(* Logix 5000 AddOnInstructionDefinition export EH_iTemp_TMT36_IOL; software revision 38.00 *)

TYPE EH_CommAOI_Data :
STRUCT
   Device_Comm_Error : BOOL;
   CommSuccess : BOOL;
   CommFailed : BOOL;
   CommTimeOut : BOOL;
   StateDone : BOOL;
   NewState : BOOL;
   OldState : SINT;
   PortSize : SINT;
   DevicePort : SINT;
   MaxState : SINT;
   State : SINT;
   VendorID : INT;
   DeviceID : DINT;
   CyclicData : INT[16];
   AcyclicData : DINT[8];
   ReplayIndex : INT;
   AOI_Diagnostic : DINT;
   ConnectionStatus : DINT;
   OutputData : INT[16];
END_STRUCT
END_TYPE

ADD_ON_INSTRUCTION EH_iTemp_TMT36_IOL   (* revision 1.1, vendor Endress+Hauser *)
// iTemp TMT36 Rev 1 IO-Link
// Revision note:
// 1.1 Changed the Datatype from Unsigned to Signed
// Add Disconnect check
VAR_IN_OUT
   DataToSend : INT[10]; {required}
   CommAOIBusy : DINT; {required}
   ActiveComPort : DINT; {required}
   DeviceAOISendRequest : DINT; {required}
   CommError : INT; {required}
   DeviceData : EH_CommAOI_Data; {required}
END_VAR
VAR_INPUT
   iSetSimulation : BOOL; {visible}
   iSimulationVariable : INT; {visible}
   iSimulationValue : REAL; {visible}
   iSetUnit : BOOL; {visible}
   iUnit : SINT; {visible}
   iParameterizeSetpoints : BOOL; {visible}
   iSSC1_SetPoint1 : REAL; {visible}
   iSSC1_SetPoint2 : REAL; {visible}
   iSSC1_Logic : SINT; {visible}
   iSSC1_Mode : SINT; {visible}
   iSSC1_Hysteresis : REAL; {visible}
   iSSC2_SetPoint1 : REAL; {visible}
   iSSC2_SetPoint2 : REAL; {visible}
   iSSC2_Logic : SINT; {visible}
   iSSC2_Mode : SINT; {visible}
   iSSC2_Hysteresis : REAL; {visible}
   iTeachSSC1 : BOOL; {visible}
   iSelectSP_SSC1 : SINT; {visible}
   iTeachSSC2 : BOOL; {visible}
   iSelectSP_SSC2 : SINT; {visible}
END_VAR
VAR_OUTPUT
   qVendor_ID : DINT; {access Read Only, visible}
   qDevice_ID : DINT; {access Read Only, visible}
   qTemperature : REAL; {visible}
   qExtendedDeviceStatus : INT; {access Read Only, visible}
   qSSC_1 : BOOL; {access Read Only, visible}
   qSSC1_SetPoint1 : REAL; {access Read Only, visible}
   qSSC1_SetPoint2 : REAL; {access Read Only, visible}
   qSSC_2 : BOOL; {access Read Only, visible}
   qSSC2_SetPoint1 : REAL; {access Read Only, visible}
   qSSC2_SetPoint2 : REAL; {access Read Only, visible}
   qUnit : DINT; {access Read Only, visible}
   qAOI_Diagnostic : DINT; {access Read Only, visible}
END_VAR
VAR_IN_OUT
   qAOI_Diagnostic_String : STRING; {required}
END_VAR
VAR_OUTPUT
   qActual_Diagnostics_Code : DINT; {access Read Only, visible}
END_VAR
VAR_IN_OUT
   qActual_Diagnostics_String : STRING; {required}
END_VAR
VAR_OUTPUT
   qLast_Diagnostics_Code : DINT; {visible}
END_VAR
VAR_IN_OUT
   qLast_Diagnostics_String : STRING; {required}
END_VAR
VAR_OUTPUT
   qCommError : DINT; {access None}
   qCommunicationBusy : DINT; {access Read Only, visible}
   qDeviceConnectionError : BOOL; {access Read Only, visible}
END_VAR
VAR
   Cond_DINT : DINT; {access None}
   Temp_DINT : DINT; {access None}
   Calc_Temperature : DINT; {access None}
   CMD_Index : INT; {access None}
   CMD_Subindex : INT; {access None}
   CMD_ByteLength : INT; {access None}
   oldCondStatus : INT; {access None}
   SetSimulation : SINT; {access None}
   SetTotalizer : SINT; {access None}
   oldSetSimulation : SINT; {access None}
   oldSetUnit : SINT; {access None}
   Trigger : BOOL; {access None}
   CMD_Rd : BOOL; {access None}
   CMD_Wr : BOOL; {access None}
   SimulationDINT : DINT; {access None}
   SimulationReal : DINT; {access None}
   Pressure_DINT : DINT; {access None}
   Level_DINT : DINT; {access None}
   InputByteLength : DINT; {access None}
   AOI_Prio : BOOL; {access None}
   ActiveAOI : BOOL; {access None}
   StateMin : DINT; {access None}
   firstTimeDone : BOOL; {access None}
   NextStep : BOOL; {access None}
   OldStatus : DINT; {access None}
   ChangedStatus : BOOL; {access None}
   CondStatusChanged : BOOL; {access None}
   Calc_ExtendedDeviceStatus : DINT; {access None}
   MassFlow_DINT : DINT; {access None}
   Density_DINT : DINT; {access None}
   oldParameterize : SINT; {access None}
   Parameterize : SINT; {access None}
   TeachSSC1Trigger : SINT; {access None}
   TeachSSC2Trigger : SINT; {access None}
   SimChanged : BOOL; {access None}
   Skip : BOOL; {access None}
   CondStatusActive : BOOL; {access None}
   SimActive : BOOL; {access None}
   DeviceID : DINT; {access None}
   FALSE : BOOL; {access None}
   TRUE : BOOL := 1; {access None}
   temp_string1 : STRING; {access None}
   temp_string2 : STRING; {access None}
   oldTeachSSC2Trigger : SINT; {access None}
   oldTeachSSC1Trigger : SINT; {access None}
   SetUnit : SINT; {access None}
   ParameterizeChanged : BOOL; {access None}
   ParameterizeActive : BOOL; {access None}
   TempAcyclic_DINT : DINT; {access None}
   TeachSSC2TriggerChanged : BOOL; {access None}
   TeachSSC1TriggerChanged : BOOL; {access None}
   TeachSSC1TriggerActive : BOOL; {access None}
   TeachSSC2TriggerActive : BOOL; {access None}
   StandardTimer : FBD_TIMER; {access None}
   qTemperatureTEMP : REAL; {access None}
   init : BOOL; {access None}
   UnitChanged : BOOL; {access None}
   UnitActive : BOOL; {access None}
END_VAR

ROUTINE Logic   (* structured text *)
// Picomag Communication via AL1323
   // =======================================================================
   // Endress+Hauser Digital Solutions
   // ©Copyright (2024) All Rights Reserved
   // =======================================================================
   // Name:                EH_iTemp_TMT36_IOL
   // Version:             1.1
   // Datum:               11.2025
   // Library:             01.01.00
   // Engineering:         Studio5000 V38.00.00
   // Author:              EH
   // =======================================================================
   
   qAOI_Diagnostic := DeviceData.AOI_Diagnostic;
   qCommunicationBusy := CommAOIBusy;
   DeviceID := 9698817;
   StateMin := 0;
   DeviceData.MaxState := 98;
   
   if DeviceData.DevicePort = 0 or DeviceData.DeviceID <> DeviceID or DeviceData.ConnectionStatus <> 1 then
   
   	qVendor_ID := DeviceData.VendorID;
   	qDevice_ID := DeviceData.DeviceID;
   	qTemperature	:= 0;
   	qExtendedDeviceStatus	:= 0;
   	qSSC_1	:= 0;
   	qSSC1_SetPoint1	:= 0;
   	qSSC1_SetPoint2	:= 0;
   	qSSC_2	:= 0;
   	qSSC2_SetPoint1	:= 0;
   	qSSC2_SetPoint2	:= 0;
   	qUnit := 0;
   	qActual_Diagnostics_Code	:= 0;
   	qLast_Diagnostics_Code	:= 0;
   	qLast_Diagnostics_String	:= '';
   	oldCondStatus := 0;
   	CondStatusChanged := FALSE;
   	init := FALSE;
   
   	if DeviceData.DevicePort = 0 then
   
   		qActual_Diagnostics_String	:= 'Device Port is Zero';
   		DeviceData.AOI_Diagnostic.1 := TRUE;
   
   	elsif DeviceData.ConnectionStatus <> 1 then
   
   		qActual_Diagnostics_String	:= 'No Device connected';
   		qDeviceConnectionError := TRUE;
   
   	elsif DeviceData.DeviceID <> DeviceID then
   
   		qActual_Diagnostics_String	:= 'Wrong DeviceID';
   		DeviceData.AOI_Diagnostic.2 := TRUE;
   	end_if;
   
   else
   
   	if qActual_Diagnostics_Code = 0  then
   
   		qActual_Diagnostics_String	:= '--------';
   
   	end_if;
   
   	if qLast_Diagnostics_Code = 0 then
   
   		qLast_Diagnostics_String	:= '--------';
   
   	end_if;
   
   	DeviceData.AOI_Diagnostic.1 := FALSE;
   	qDeviceConnectionError := FALSE;
   	DeviceData.AOI_Diagnostic.2  := FALSE;
   
   end_if;
   
   // Case device disconnected during communication to avoid blocking the communication
   if (DeviceData.AOI_Diagnostic.0 or qDeviceConnectionError or DeviceData.AOI_Diagnostic.2) and ActiveAOI and ActiveComPort = DeviceData.DevicePort and CommAOIBusy = 1 then
   
   	DeviceData.State := 0;
   	CommAOIBusy := 0;
   	DeviceAOISendRequest.[DeviceData.DevicePort] := 0;
   	ActiveComPort := 0;
   	ActiveAOI := 0;
   	DataToSend[0] := 0;
   	DataToSend[1] := 0;
   	DataToSend[2] := 0;
   	DataToSend[3] := 0;
   	DataToSend[4] := 0;
   	DataToSend[5] := 0;
   	DataToSend[6] := 0;
   	DataToSend[7] := 0;
   	DataToSend[8] := 0;
   	DataToSend[9] := 0;
   	DeviceData.StateDone := FALSE;
   	DeviceData.NewState := FALSE;
   	DeviceData.OldState := 0;
   	ActiveAOI := FALSE;
   
   end_if;
   
   if not DeviceData.AOI_Diagnostic.0
   	and not qDeviceConnectionError
   	and not DeviceData.AOI_Diagnostic.2
   	and DeviceData.DevicePort > 0 then
   
   	//*********************************
   	//Vendor ID
   	//*********************************
   
   		qVendor_ID := DeviceData.VendorID;
   
   	//*********************************
   	//Device ID
   	//*********************************
   
   		qDevice_ID := DeviceData.DeviceID;
   
   	//*********************************
   	// TMT36 Cyclic Input
   	//*********************************
   
   		Calc_Temperature			:= 0;
   		Calc_ExtendedDeviceStatus	:= 2;
   
   	//*********************************
   	//Process Data Temperature
   	//*********************************
   
   		Temp_DINT	 := DeviceData.CyclicData[Calc_Temperature+1];
   		Temp_DINT.8	 := DeviceData.CyclicData[Calc_Temperature+1].8;
   		Temp_DINT.9  := DeviceData.CyclicData[Calc_Temperature+1].9;
   		Temp_DINT.10 := DeviceData.CyclicData[Calc_Temperature+1].10;
   		Temp_DINT.11 := DeviceData.CyclicData[Calc_Temperature+1].11;
   		Temp_DINT.12 := DeviceData.CyclicData[Calc_Temperature+1].12;
   		Temp_DINT.13 := DeviceData.CyclicData[Calc_Temperature+1].13;
   		Temp_DINT.14 := DeviceData.CyclicData[Calc_Temperature+1].14;
   		Temp_DINT.15 := DeviceData.CyclicData[Calc_Temperature+1].15;
   		Temp_DINT.16 := DeviceData.CyclicData[Calc_Temperature].0;
   		Temp_DINT.17 := DeviceData.CyclicData[Calc_Temperature].1;
   		Temp_DINT.18 := DeviceData.CyclicData[Calc_Temperature].2;
   		Temp_DINT.19 := DeviceData.CyclicData[Calc_Temperature].3;
   		Temp_DINT.20 := DeviceData.CyclicData[Calc_Temperature].4;
   		Temp_DINT.21 := DeviceData.CyclicData[Calc_Temperature].5;
   		Temp_DINT.22 := DeviceData.CyclicData[Calc_Temperature].6;
   		Temp_DINT.23 := DeviceData.CyclicData[Calc_Temperature].7;
   		Temp_DINT.24 := DeviceData.CyclicData[Calc_Temperature].8;
   		Temp_DINT.25 := DeviceData.CyclicData[Calc_Temperature].9;
   		Temp_DINT.26 := DeviceData.CyclicData[Calc_Temperature].10;
   		Temp_DINT.27 := DeviceData.CyclicData[Calc_Temperature].11;
   		Temp_DINT.28 := DeviceData.CyclicData[Calc_Temperature].12;
   		Temp_DINT.29 := DeviceData.CyclicData[Calc_Temperature].13;
   		Temp_DINT.30 := DeviceData.CyclicData[Calc_Temperature].14;
   		Temp_DINT.31 := DeviceData.CyclicData[Calc_Temperature].15;
   
   		COP(Temp_DINT,qTemperatureTEMP,1);
   
   		// Unit of the process value, 32 = °C, 33 = °F
   		if qUnit = 33 then
   
   			qTemperature := (qTemperatureTEMP * 1.8) +32;
   
   		else
   
   			qTemperature := qTemperatureTEMP;
   
   		end_if;
   
   
   	//*********************************
   	// Extended device Status
   	//*********************************
   
   		qExtendedDeviceStatus.0 := DeviceData.CyclicData[Calc_ExtendedDeviceStatus].8;
   		qExtendedDeviceStatus.1 := DeviceData.CyclicData[Calc_ExtendedDeviceStatus].9;
   		qExtendedDeviceStatus.2 := DeviceData.CyclicData[Calc_ExtendedDeviceStatus].10;
   		qExtendedDeviceStatus.3 := DeviceData.CyclicData[Calc_ExtendedDeviceStatus].11;
   		qExtendedDeviceStatus.4 := DeviceData.CyclicData[Calc_ExtendedDeviceStatus].12;
   		qExtendedDeviceStatus.5 := DeviceData.CyclicData[Calc_ExtendedDeviceStatus].13;
   		qExtendedDeviceStatus.6 := DeviceData.CyclicData[Calc_ExtendedDeviceStatus].14;
   		qExtendedDeviceStatus.7 := DeviceData.CyclicData[Calc_ExtendedDeviceStatus].15;
   
   	//*********************************
   	// Process Parameter SSC
   	//*********************************
   
   		qSSC_1 := DeviceData.CyclicData[Calc_ExtendedDeviceStatus].0;
   		qSSC_2 := DeviceData.CyclicData[Calc_ExtendedDeviceStatus].1;
   
   	//*********************************
   	// Checking for Changed Status @ Input or Condenced Status
   	//*********************************
   
   	SetSimulation.0 := iSetSimulation;
   	Parameterize.0 := iParameterizeSetpoints;
   	TeachSSC1Trigger.0 := iTeachSSC1;
   	TeachSSC2Trigger.0 := iTeachSSC2;
   	SetUnit.0 := iSetUnit;
   
   	if oldCondStatus <> qExtendedDeviceStatus and not CondStatusChanged then
   
   		CondStatusChanged := TRUE;
   		oldCondStatus := qExtendedDeviceStatus;
   
   	end_if;
   
   	if oldSetSimulation <> SetSimulation and not SimChanged then
   
   		if oldSetSimulation < SetSimulation then
   
   			SimChanged := TRUE;
   
   		end_if;
   
   		oldSetSimulation := SetSimulation;
   
   	end_if;
   
   	if oldSetUnit <> SetUnit and not UnitChanged then
   
   		if oldSetUnit < SetUnit then
   
   			UnitChanged := TRUE;
   
   		end_if;
   
   		oldSetUnit := SetUnit;
   
   	end_if;
   
   	if oldParameterize <> Parameterize and not ParameterizeChanged then
   
   		if oldParameterize < Parameterize then
   
   			ParameterizeChanged := TRUE;
   
   		end_if;
   
   		oldParameterize := Parameterize;
   
   	end_if;
   
   	if oldTeachSSC1Trigger <> TeachSSC1Trigger and not TeachSSC1TriggerChanged then
   
   		if oldTeachSSC1Trigger < TeachSSC1Trigger then
   
   			TeachSSC1TriggerChanged := TRUE;
   
   		end_if;
   
   		oldTeachSSC1Trigger := TeachSSC1Trigger;
   
   	end_if;
   
   	if oldTeachSSC2Trigger <> TeachSSC2Trigger and not TeachSSC2TriggerChanged then
   
   		if oldTeachSSC2Trigger < TeachSSC2Trigger then
   
   			TeachSSC2TriggerChanged := TRUE;
   
   		end_if;
   
   		oldTeachSSC2Trigger := TeachSSC2Trigger;
   
   	end_if;
   
   	if CondStatusChanged
   	and not ActiveAOI
   	and not CondStatusActive
   	and not Skip then
   
   		DeviceAOISendRequest.[DeviceData.DevicePort] := TRUE;
   		CondStatusActive := TRUE;
   		Skip := TRUE;
   
   	elsif SimChanged
   		and not ActiveAOI
   		and not SimActive
   		and not Skip then
   
   		DeviceAOISendRequest.[DeviceData.DevicePort] := TRUE;
   		SimActive := TRUE;
   		Skip := TRUE;
   
   	elsif UnitChanged
   		and not ActiveAOI
   		and not UnitActive
   		and not Skip then
   
   		DeviceAOISendRequest.[DeviceData.DevicePort] := TRUE;
   		UnitActive := TRUE;
   		Skip := TRUE;
   
   	elsif TeachSSC1TriggerChanged
   		and not ActiveAOI
   		and not TeachSSC1TriggerActive
   		and not Skip then
   
   		DeviceAOISendRequest.[DeviceData.DevicePort] := TRUE;
   		TeachSSC1TriggerActive := TRUE;
   		Skip := TRUE;
   
   	elsif TeachSSC2TriggerChanged
   		and not ActiveAOI
   		and not TeachSSC2TriggerActive
   		and not Skip then
   
   		DeviceAOISendRequest.[DeviceData.DevicePort] := TRUE;
   		TeachSSC2TriggerActive := TRUE;
   		Skip := TRUE;
   
   	elsif ParameterizeChanged
   		and not ActiveAOI
   		and not ParameterizeActive
   		and not Skip then
   
   		DeviceAOISendRequest.[DeviceData.DevicePort] := TRUE;
   		ParameterizeActive := TRUE;
   		Skip := TRUE;
   
   	end_if;
   
   	if ActiveComPort = DeviceData.DevicePort then
   
   		AOI_Prio := TRUE;
   
   	else
   
   		AOI_Prio := FALSE;
   
   	end_if;
   
   	if (SimActive or UnitActive or TeachSSC1TriggerActive or TeachSSC2TriggerActive or ParameterizeActive or CondStatusActive) and CommAOIBusy = 1  and DeviceData.State = 0 and AOI_Prio and not ActiveAOI then
   
   		ActiveAOI := TRUE;
   		Skip := FALSE;
   
   	end_if;
   
   	qCommunicationBusy := CommAOIBusy;
   	qAOI_Diagnostic :=DeviceData.AOI_Diagnostic;
   
   	//*********************************
   	// States for Execution
   	//*********************************
   
   	if ActiveAOI or DeviceData.State = DeviceData.MaxState then
   
   	case DeviceData.State of
   
   		//*********************************
   		0: // Start
   		//*********************************
   
   			Trigger := FALSE;
   			CMD_Index := 0;
   			CMD_Subindex := 0;
   			CMD_Wr := FALSE;
   			CMD_Rd := FALSE;
   			CMD_ByteLength := 0;
   
   			if DeviceData.DevicePort = ActiveComPort then
   
   				DeviceData.CommSuccess := FALSE;
   				DeviceData.CommTimeOut := FALSE;
   				DeviceData.NewState := TRUE;
   				DeviceData.StateDone := FALSE;
   
   			end_if;
   
   			if SimActive then
   
   				DeviceData.AOI_Diagnostic := 0;
   				DeviceData.State := 1;
   
   			elsif UnitActive then
   
   				DeviceData.AOI_Diagnostic := 0;
   				DeviceData.State := 4;
   
   			elsif ParameterizeActive then
   
   				DeviceData.AOI_Diagnostic := 0;
   				DeviceData.State := 43;
   
   			elsif TeachSSC1TriggerActive then
   
   				DeviceData.AOI_Diagnostic := 0;
   				DeviceData.State := 50;
   
   			elsif TeachSSC2TriggerActive then
   
   				DeviceData.AOI_Diagnostic := 0;
   				DeviceData.State := 60;
   
   			elsif CondStatusChanged then
   
   				if not init then
   
   					DeviceData.State := 5;
   
   				else
   
   					DeviceData.State := 90;
   
   				end_if;
   
   			end_if;
   
   		//*********************************
   		1: // Set Simulation
   		//*********************************
   
   			CMD_Index := 8259;
   			CMD_Subindex := 0;
   			CMD_Wr := TRUE;	// Only Read or Write can be active
   			CMD_Rd := FALSE;
   			CMD_ByteLength := 1;	//Check Length
   			DataToSend[6]:= 0;
   			DataToSend[7]:= 0;
   
   			// 0 = Off, 1 = Temperature
   			DataToSend[6].0 := iSimulationVariable.0;
   			DataToSend[6].1 := iSimulationVariable.1;
   			DataToSend[6].2 := iSimulationVariable.2;
   			DataToSend[6].3 := iSimulationVariable.3;
   			DataToSend[6].4 := iSimulationVariable.4;
   			DataToSend[6].5 := iSimulationVariable.5;
   			DataToSend[6].6 := iSimulationVariable.6;
   			DataToSend[6].7 := iSimulationVariable.7;
   
   			Trigger := TRUE;
   
   			if DeviceData.NewState then
   
   				DeviceData.StateDone := TRUE;
   
   			end_if;
   
   			if  DeviceData.CommSuccess and DeviceData.ReplayIndex = CMD_Index then
   
   				Trigger := FALSE;
   				DeviceData.OldState := DeviceData.State;
   				DeviceData.State := DeviceData.State + 1;
   				DeviceData.CommSuccess := FALSE;
   				DeviceData.AcyclicData[0] := 0;
   				DeviceData.NewState := TRUE;
   
   			elsif DeviceData.CommTimeOut then
   
   				temp_string1 := 'Error in step ';
   				Temp_DINT := DeviceData.State;
   				DTOS(Temp_DINT, temp_string2);
   				CONCAT(temp_string1, temp_string2, qAOI_Diagnostic_String);
   
   				DeviceData.OldState := DeviceData.State;
   				DeviceData.State := DeviceData.MaxState;
   				DeviceData.CommTimeOut := FALSE;
   				DeviceData.AcyclicData[0] := 0;
   				DeviceData.NewState := TRUE;
   
   			end_if;
   
   
   		//*********************************
   		2: // Set Simulation Value
   		//*********************************
   
   			CMD_Index := 8254;
   			CMD_Subindex := 0;
   			CMD_Wr := TRUE;
   			CMD_Rd := FALSE;
   			CMD_ByteLength := 4;
   			DataToSend[6]:= 0;
   			DataToSend[7]:= 0;
   
   		 	COP(iSimulationValue,SimulationDINT,1);		// Copy the Bits from the Real in a DINT
   
   			DataToSend[6].0 :=  SimulationDINT.24;
   			DataToSend[6].1 :=  SimulationDINT.25;
   			DataToSend[6].2 :=  SimulationDINT.26;
   			DataToSend[6].3 :=  SimulationDINT.27;
   			DataToSend[6].4 :=  SimulationDINT.28;
   			DataToSend[6].5 :=  SimulationDINT.29;
   			DataToSend[6].6 :=  SimulationDINT.30;
   			DataToSend[6].7 :=  SimulationDINT.31;
   			DataToSend[6].8 :=  SimulationDINT.16;
   			DataToSend[6].9 :=  SimulationDINT.17;
   			DataToSend[6].10 := SimulationDINT.18;
   			DataToSend[6].11 := SimulationDINT.19;
   			DataToSend[6].12 := SimulationDINT.20;
   			DataToSend[6].13 := SimulationDINT.21;
   			DataToSend[6].14 := SimulationDINT.22;
   			DataToSend[6].15 := SimulationDINT.23;
   			DataToSend[7].0  := SimulationDINT.8;
   			DataToSend[7].1  := SimulationDINT.9;
   			DataToSend[7].2  := SimulationDINT.10;
   			DataToSend[7].3  := SimulationDINT.11;
   			DataToSend[7].4  := SimulationDINT.12;
   			DataToSend[7].5  := SimulationDINT.13;
   			DataToSend[7].6  := SimulationDINT.14;
   			DataToSend[7].7  := SimulationDINT.15;
   			DataToSend[7].8  := SimulationDINT.0;
   			DataToSend[7].9  := SimulationDINT.1;
   			DataToSend[7].10 := SimulationDINT.2;
   			DataToSend[7].11 := SimulationDINT.3;
   			DataToSend[7].12 := SimulationDINT.4;
   			DataToSend[7].13 := SimulationDINT.5;
   			DataToSend[7].14 := SimulationDINT.6;
   			DataToSend[7].15 := SimulationDINT.7;
   
   			Trigger := TRUE;
   
   			if DeviceData.NewState then
   
   				DeviceData.StateDone := TRUE;
   
   			end_if;
   
   			if DeviceData.CommSuccess and DeviceData.ReplayIndex = CMD_Index then
   
   				Trigger := FALSE;
   				DeviceData.OldState := DeviceData.State;
   				DeviceData.State := DeviceData.MaxState;
   				DeviceData.CommSuccess := FALSE;
   				DeviceData.AcyclicData[0] := 0;
   				DeviceData.NewState := TRUE;
   
   			elsif DeviceData.CommTimeOut then
   
   				temp_string1 := 'Error in step ';
   				Temp_DINT := DeviceData.State;
   				DTOS(Temp_DINT, temp_string2);
   				CONCAT(temp_string1, temp_string2, qAOI_Diagnostic_String);
   
   				DeviceData.OldState := DeviceData.State;
   				DeviceData.State := DeviceData.MaxState;	//Check State
   				DeviceData.CommTimeOut := FALSE;
   				DeviceData.AcyclicData[0] := 0;
   				DeviceData.NewState := TRUE;
   
   			end_if;
   
   		//*********************************
   		4: // Set Unit
   		//*********************************
   
   			CMD_Index := 8274;
   			CMD_Subindex := 0;
   			CMD_Wr := TRUE;								// Only Read or Write can be active = 1
   			CMD_Rd := FALSE;
   			CMD_ByteLength := 1;
   			DataToSend[6] := 0;
   			DataToSend[7] := 0;
   
   			if iUnit = 32 OR iUnit = 33 then
   
   				DataToSend[6].0 := iUnit.0;
   				DataToSend[6].1 := iUnit.1;
   				DataToSend[6].2 := iUnit.2;
   				DataToSend[6].3 := iUnit.3;
   				DataToSend[6].4 := iUnit.4;
   				DataToSend[6].5 := iUnit.5;
   				DataToSend[6].6 := iUnit.6;
   				DataToSend[6].7 := iUnit.7;
   				Trigger := TRUE;
   
   				if DeviceData.NewState then
   					DeviceData.StateDone := TRUE;
   				end_if;
   
   				if  DeviceData.CommSuccess and DeviceData.ReplayIndex = CMD_Index then
   
   					Trigger := FALSE;
   					DeviceData.OldState := DeviceData.State;
   					DeviceData.State := DeviceData.State + 1;
   					DeviceData.CommSuccess := FALSE;
   					DeviceData.AcyclicData[0] := 0;
   					DeviceData.NewState := TRUE;
   
   			 	elsif DeviceData.CommTimeOut then
   
   					temp_string1 := 'Error in step ';
   					Temp_DINT := DeviceData.State;
   					DTOS(Temp_DINT, temp_string2);
   					CONCAT(temp_string1, temp_string2, qAOI_Diagnostic_String);
   
   					DeviceData.OldState := DeviceData.State;
   					DeviceData.State := DeviceData.MaxState;	//Check State
   					DeviceData.CommTimeOut := FALSE;
   					DeviceData.AcyclicData[0] := 0;
   					DeviceData.NewState := TRUE;
   
   				end_if;
   
   			else
   
   					temp_string1 := 'Error in step ';
   					Temp_DINT := DeviceData.State;
   					DTOS(Temp_DINT, temp_string2);
   					CONCAT(temp_string1, temp_string2, qAOI_Diagnostic_String);
   
   					DeviceData.OldState := DeviceData.State;
   					DeviceData.State := DeviceData.MaxState;
   					DeviceData.CommTimeOut := FALSE;
   					DeviceData.AcyclicData[0] := 0;
   					DeviceData.NewState := TRUE;
   
   	        end_if;
   
   
   		//*********************************
   		5: // Read Unit
   		//*********************************
   
   				CMD_Index := 8274;
   				CMD_Subindex := 0;
   				CMD_Wr := FALSE;
   				CMD_Rd := TRUE;
   				CMD_ByteLength := 1;
   				Trigger := TRUE;
   
   				if DeviceData.NewState then
   					DeviceData.StateDone := TRUE;
   				end_if;
   
   				if  DeviceData.CommSuccess and DeviceData.ReplayIndex = CMD_Index then
   
   					qUnit.0	:= DeviceData.AcyclicData[0].0;
   					qUnit.1	:= DeviceData.AcyclicData[0].1;
   					qUnit.2	:= DeviceData.AcyclicData[0].2;
   					qUnit.3	:= DeviceData.AcyclicData[0].3;
   					qUnit.4	:= DeviceData.AcyclicData[0].4;
   					qUnit.5	:= DeviceData.AcyclicData[0].5;
   					qUnit.6	:= DeviceData.AcyclicData[0].6;
   					qUnit.7	:= DeviceData.AcyclicData[0].7;
   
   					Trigger := FALSE;
   					DeviceData.OldState := DeviceData.State;
   					DeviceData.State := DeviceData.MaxState;
   					DeviceData.CommSuccess := FALSE;
   					DeviceData.AcyclicData[0] := 0;
   					DeviceData.NewState := TRUE;
   
   					if not init then
   
   						init := TRUE;
   						DeviceData.State := 90;
   
   					end_if;
   
   				 elsif DeviceData.CommTimeOut then
   
   					temp_string1 := 'Error in step ';
   					Temp_DINT := DeviceData.State;
   					DTOS(Temp_DINT, temp_string2);
   					CONCAT(temp_string1, temp_string2, qAOI_Diagnostic_String);
   
   					DeviceData.OldState := DeviceData.State;
   					DeviceData.State := DeviceData.MaxState;
   					DeviceData.CommTimeOut := FALSE;
   					DeviceData.AcyclicData[0] := 0;
   					DeviceData.NewState := TRUE;
   
   				end_if;
   
   
   		//************************************
   		43: // SSC1 Setpoint - SSC1 param
   		//************************************
   
   			CMD_Index := 60;
   			CMD_Subindex := 0;
   			CMD_Wr := TRUE;
   			CMD_Rd := FALSE;
   			CMD_ByteLength := 8;
   			DataToSend[6]:= 0;
   			DataToSend[7]:= 0;
   			DataToSend[8]:= 0;
   			DataToSend[9]:= 0;
   
   		 	COP(iSSC1_SetPoint1,SimulationDINT,1);		// Copy the Bits from the Real in a DINT
   
   			DataToSend[6].0 :=  SimulationDINT.24;
   			DataToSend[6].1 :=  SimulationDINT.25;
   			DataToSend[6].2 :=  SimulationDINT.26;
   			DataToSend[6].3 :=  SimulationDINT.27;
   			DataToSend[6].4 :=  SimulationDINT.28;
   			DataToSend[6].5 :=  SimulationDINT.29;
   			DataToSend[6].6 :=  SimulationDINT.30;
   			DataToSend[6].7 :=  SimulationDINT.31;
   			DataToSend[6].8 :=  SimulationDINT.16;
   			DataToSend[6].9 :=  SimulationDINT.17;
   			DataToSend[6].10 := SimulationDINT.18;
   			DataToSend[6].11 := SimulationDINT.19;
   			DataToSend[6].12 := SimulationDINT.20;
   			DataToSend[6].13 := SimulationDINT.21;
   			DataToSend[6].14 := SimulationDINT.22;
   			DataToSend[6].15 := SimulationDINT.23;
   			DataToSend[7].0  := SimulationDINT.8;
   			DataToSend[7].1  := SimulationDINT.9;
   			DataToSend[7].2  := SimulationDINT.10;
   			DataToSend[7].3  := SimulationDINT.11;
   			DataToSend[7].4  := SimulationDINT.12;
   			DataToSend[7].5  := SimulationDINT.13;
   			DataToSend[7].6  := SimulationDINT.14;
   			DataToSend[7].7  := SimulationDINT.15;
   			DataToSend[7].8  := SimulationDINT.0;
   			DataToSend[7].9  := SimulationDINT.1;
   			DataToSend[7].10 := SimulationDINT.2;
   			DataToSend[7].11 := SimulationDINT.3;
   			DataToSend[7].12 := SimulationDINT.4;
   			DataToSend[7].13 := SimulationDINT.5;
   			DataToSend[7].14 := SimulationDINT.6;
   			DataToSend[7].15 := SimulationDINT.7;
   
   			COP(iSSC1_SetPoint2,SimulationDINT,1);		// Copy the Bits from the Real in a DINT
   
   			DataToSend[8].0 :=  SimulationDINT.24;
   			DataToSend[8].1 :=  SimulationDINT.25;
   			DataToSend[8].2 :=  SimulationDINT.26;
   			DataToSend[8].3 :=  SimulationDINT.27;
   			DataToSend[8].4 :=  SimulationDINT.28;
   			DataToSend[8].5 :=  SimulationDINT.29;
   			DataToSend[8].6 :=  SimulationDINT.30;
   			DataToSend[8].7 :=  SimulationDINT.31;
   			DataToSend[8].8 :=  SimulationDINT.16;
   			DataToSend[8].9 :=  SimulationDINT.17;
   			DataToSend[8].10 := SimulationDINT.18;
   			DataToSend[8].11 := SimulationDINT.19;
   			DataToSend[8].12 := SimulationDINT.20;
   			DataToSend[8].13 := SimulationDINT.21;
   			DataToSend[8].14 := SimulationDINT.22;
   			DataToSend[8].15 := SimulationDINT.23;
   			DataToSend[9].0  := SimulationDINT.8;
   			DataToSend[9].1  := SimulationDINT.9;
   			DataToSend[9].2  := SimulationDINT.10;
   			DataToSend[9].3  := SimulationDINT.11;
   			DataToSend[9].4  := SimulationDINT.12;
   			DataToSend[9].5  := SimulationDINT.13;
   			DataToSend[9].6  := SimulationDINT.14;
   			DataToSend[9].7  := SimulationDINT.15;
   			DataToSend[9].8  := SimulationDINT.0;
   			DataToSend[9].9  := SimulationDINT.1;
   			DataToSend[9].10 := SimulationDINT.2;
   			DataToSend[9].11 := SimulationDINT.3;
   			DataToSend[9].12 := SimulationDINT.4;
   			DataToSend[9].13 := SimulationDINT.5;
   			DataToSend[9].14 := SimulationDINT.6;
   			DataToSend[9].15 := SimulationDINT.7;
   			Trigger := TRUE;
   
   			if DeviceData.NewState then
   
   				DeviceData.StateDone := TRUE;
   
   			end_if;
   
   			if DeviceData.CommSuccess and DeviceData.ReplayIndex = CMD_Index then
   
   				Trigger := FALSE;
   				DeviceData.OldState := DeviceData.State;
   				DeviceData.State := DeviceData.State + 1;
   				DeviceData.CommSuccess := FALSE;
   				DeviceData.AcyclicData[0] := 0;
   				DeviceData.NewState := TRUE;
   
   			elsif DeviceData.CommTimeOut then
   
   				temp_string1 := 'Error in step ';
   				Temp_DINT := DeviceData.State;
   				DTOS(Temp_DINT, temp_string2);
   				CONCAT(temp_string1, temp_string2, qAOI_Diagnostic_String);
   
   				DeviceData.OldState := DeviceData.State;
   				DeviceData.State := DeviceData.MaxState;	//Check State
   				DeviceData.CommTimeOut := FALSE;
   				DeviceData.AcyclicData[0] := 0;
   				DeviceData.NewState := TRUE;
   
   			end_if;
   
   
   		//********************************************
   		44: // SSC1 config / Logic & Mode & Hysteresis
   		//********************************************
   
   			CMD_Index := 61;
   			CMD_Subindex := 0;
   			CMD_Wr := TRUE;
   			CMD_Rd := FALSE;
   			CMD_ByteLength := 6;
   			DataToSend[6]:= 0;
   			DataToSend[7]:= 0;
   			DataToSend[8]:= 0;
   
   			// 0 = High active, 1 = Low active
   			DataToSend[6].0 :=  iSSC1_Logic.0;
   			DataToSend[6].1 :=  iSSC1_Logic.1;
   			DataToSend[6].2 :=  iSSC1_Logic.2;
   			DataToSend[6].3 :=  iSSC1_Logic.3;
   			DataToSend[6].4 :=  iSSC1_Logic.4;
   			DataToSend[6].5 :=  iSSC1_Logic.5;
   			DataToSend[6].6 :=  iSSC1_Logic.6;
   			DataToSend[6].7 :=  iSSC1_Logic.7;
   
   			// Logic of the switch output 1, 0 = Deactivated, 1 = Single point, 2 = Window, 3 = Two point
   			DataToSend[6].8 :=  iSSC1_Mode.0;
   			DataToSend[6].9 :=  iSSC1_Mode.1;
   			DataToSend[6].10 := iSSC1_Mode.2;
   			DataToSend[6].11 := iSSC1_Mode.3;
   			DataToSend[6].12 := iSSC1_Mode.4;
   			DataToSend[6].13 := iSSC1_Mode.5;
   			DataToSend[6].14 := iSSC1_Mode.6;
   			DataToSend[6].15 := iSSC1_Mode.7;
   
   			// Hysteresis of the switch output
   		 	COP(iSSC1_Hysteresis,SimulationDINT,1);		// Copy the Bits from the Real in a DINT
   
   			DataToSend[7].0 :=  SimulationDINT.24;
   			DataToSend[7].1 :=  SimulationDINT.25;
   			DataToSend[7].2 :=  SimulationDINT.26;
   			DataToSend[7].3 :=  SimulationDINT.27;
   			DataToSend[7].4 :=  SimulationDINT.28;
   			DataToSend[7].5 :=  SimulationDINT.29;
   			DataToSend[7].6 :=  SimulationDINT.30;
   			DataToSend[7].7 :=  SimulationDINT.31;
   			DataToSend[7].8 :=  SimulationDINT.16;
   			DataToSend[7].9 :=  SimulationDINT.17;
   			DataToSend[7].10 := SimulationDINT.18;
   			DataToSend[7].11 := SimulationDINT.19;
   			DataToSend[7].12 := SimulationDINT.20;
   			DataToSend[7].13 := SimulationDINT.21;
   			DataToSend[7].14 := SimulationDINT.22;
   			DataToSend[7].15 := SimulationDINT.23;
   			DataToSend[8].0  := SimulationDINT.8;
   			DataToSend[8].1  := SimulationDINT.9;
   			DataToSend[8].2  := SimulationDINT.10;
   			DataToSend[8].3  := SimulationDINT.11;
   			DataToSend[8].4  := SimulationDINT.12;
   			DataToSend[8].5  := SimulationDINT.13;
   			DataToSend[8].6  := SimulationDINT.14;
   			DataToSend[8].7  := SimulationDINT.15;
   			DataToSend[8].8  := SimulationDINT.0;
   			DataToSend[8].9  := SimulationDINT.1;
   			DataToSend[8].10 := SimulationDINT.2;
   			DataToSend[8].11 := SimulationDINT.3;
   			DataToSend[8].12 := SimulationDINT.4;
   			DataToSend[8].13 := SimulationDINT.5;
   			DataToSend[8].14 := SimulationDINT.6;
   			DataToSend[8].15 := SimulationDINT.7;
   
   			Trigger := TRUE;
   
   			if DeviceData.NewState then
   
   				DeviceData.StateDone := TRUE;
   
   			end_if;
   
   			if DeviceData.CommSuccess and DeviceData.ReplayIndex = CMD_Index then
   
   				Trigger := FALSE;
   				DeviceData.OldState := DeviceData.State;
   				DeviceData.State := DeviceData.State + 1;
   				DeviceData.CommSuccess := FALSE;
   				DeviceData.AcyclicData[0] := 0;
   				DeviceData.NewState := TRUE;
   
   			elsif DeviceData.CommTimeOut then
   
   				temp_string1 := 'Error in step ';
   				Temp_DINT := DeviceData.State;
   				DTOS(Temp_DINT, temp_string2);
   				CONCAT(temp_string1, temp_string2, qAOI_Diagnostic_String);
   
   				DeviceData.OldState := DeviceData.State;
   				DeviceData.State := DeviceData.MaxState;	//Check State
   				DeviceData.CommTimeOut := FALSE;
   				DeviceData.AcyclicData[0] := 0;
   				DeviceData.NewState := TRUE;
   
   			end_if;
   
   
   		//************************************
   		45: // SSC2 Setpoint - SSC2 param
   		//************************************
   
   			CMD_Index := 62;
   			CMD_Subindex := 0;
   			CMD_Wr := TRUE;
   			CMD_Rd := FALSE;
   			CMD_ByteLength := 8;
   			DataToSend[6]:= 0;
   			DataToSend[7]:= 0;
   			DataToSend[8]:= 0;
   			DataToSend[9]:= 0;
   
   		 	COP(iSSC2_SetPoint1,SimulationDINT,1);		// Copy the Bits from the Real in a DINT
   
   			DataToSend[6].0 :=  SimulationDINT.24;
   			DataToSend[6].1 :=  SimulationDINT.25;
   			DataToSend[6].2 :=  SimulationDINT.26;
   			DataToSend[6].3 :=  SimulationDINT.27;
   			DataToSend[6].4 :=  SimulationDINT.28;
   			DataToSend[6].5 :=  SimulationDINT.29;
   			DataToSend[6].6 :=  SimulationDINT.30;
   			DataToSend[6].7 :=  SimulationDINT.31;
   			DataToSend[6].8 :=  SimulationDINT.16;
   			DataToSend[6].9 :=  SimulationDINT.17;
   			DataToSend[6].10 := SimulationDINT.18;
   			DataToSend[6].11 := SimulationDINT.19;
   			DataToSend[6].12 := SimulationDINT.20;
   			DataToSend[6].13 := SimulationDINT.21;
   			DataToSend[6].14 := SimulationDINT.22;
   			DataToSend[6].15 := SimulationDINT.23;
   			DataToSend[7].0  := SimulationDINT.8;
   			DataToSend[7].1  := SimulationDINT.9;
   			DataToSend[7].2  := SimulationDINT.10;
   			DataToSend[7].3  := SimulationDINT.11;
   			DataToSend[7].4  := SimulationDINT.12;
   			DataToSend[7].5  := SimulationDINT.13;
   			DataToSend[7].6  := SimulationDINT.14;
   			DataToSend[7].7  := SimulationDINT.15;
   			DataToSend[7].8  := SimulationDINT.0;
   			DataToSend[7].9  := SimulationDINT.1;
   			DataToSend[7].10 := SimulationDINT.2;
   			DataToSend[7].11 := SimulationDINT.3;
   			DataToSend[7].12 := SimulationDINT.4;
   			DataToSend[7].13 := SimulationDINT.5;
   			DataToSend[7].14 := SimulationDINT.6;
   			DataToSend[7].15 := SimulationDINT.7;
   
   			COP(iSSC2_SetPoint2,SimulationDINT,1);		// Copy the Bits from the Real in a DINT
   			DataToSend[8].0 :=  SimulationDINT.24;
   			DataToSend[8].1 :=  SimulationDINT.25;
   			DataToSend[8].2 :=  SimulationDINT.26;
   			DataToSend[8].3 :=  SimulationDINT.27;
   			DataToSend[8].4 :=  SimulationDINT.28;
   			DataToSend[8].5 :=  SimulationDINT.29;
   			DataToSend[8].6 :=  SimulationDINT.30;
   			DataToSend[8].7 :=  SimulationDINT.31;
   			DataToSend[8].8 :=  SimulationDINT.16;
   			DataToSend[8].9 :=  SimulationDINT.17;
   			DataToSend[8].10 := SimulationDINT.18;
   			DataToSend[8].11 := SimulationDINT.19;
   			DataToSend[8].12 := SimulationDINT.20;
   			DataToSend[8].13 := SimulationDINT.21;
   			DataToSend[8].14 := SimulationDINT.22;
   			DataToSend[8].15 := SimulationDINT.23;
   			DataToSend[9].0  := SimulationDINT.8;
   			DataToSend[9].1  := SimulationDINT.9;
   			DataToSend[9].2  := SimulationDINT.10;
   			DataToSend[9].3  := SimulationDINT.11;
   			DataToSend[9].4  := SimulationDINT.12;
   			DataToSend[9].5  := SimulationDINT.13;
   			DataToSend[9].6  := SimulationDINT.14;
   			DataToSend[9].7  := SimulationDINT.15;
   			DataToSend[9].8  := SimulationDINT.0;
   			DataToSend[9].9  := SimulationDINT.1;
   			DataToSend[9].10 := SimulationDINT.2;
   			DataToSend[9].11 := SimulationDINT.3;
   			DataToSend[9].12 := SimulationDINT.4;
   			DataToSend[9].13 := SimulationDINT.5;
   			DataToSend[9].14 := SimulationDINT.6;
   			DataToSend[9].15 := SimulationDINT.7;
   
   			Trigger := TRUE;
   
   			if DeviceData.NewState then
   
   				DeviceData.StateDone := TRUE;
   
   			end_if;
   
   			if DeviceData.CommSuccess and DeviceData.ReplayIndex = CMD_Index then
   
   				Trigger := FALSE;
   				DeviceData.OldState := DeviceData.State;
   				DeviceData.State := DeviceData.State + 1;
   				DeviceData.CommSuccess := FALSE;
   				DeviceData.AcyclicData[0] := 0;
   				DeviceData.NewState := TRUE;
   
   			elsif DeviceData.CommTimeOut then
   
   				temp_string1 := 'Error in step ';
   				Temp_DINT := DeviceData.State;
   				DTOS(Temp_DINT, temp_string2);
   				CONCAT(temp_string1, temp_string2, qAOI_Diagnostic_String);
   
   				DeviceData.OldState := DeviceData.State;
   				DeviceData.State := DeviceData.MaxState;	//Check State
   				DeviceData.CommTimeOut := FALSE;
   				DeviceData.AcyclicData[0] := 0;
   				DeviceData.NewState := TRUE;
   
   			end_if;
   
   		//********************************************
   		46: // SSC2 config / Logic & Mode & Hysteresis
   		//********************************************
   
   			CMD_Index := 63;
   			CMD_Subindex := 0;
   			CMD_Wr := TRUE;
   			CMD_Rd := FALSE;
   			CMD_ByteLength := 6;
   			DataToSend[6]:= 0;
   			DataToSend[7]:= 0;
   			DataToSend[8]:= 0;
   
   			// 0 = High active, 1 = Low active
   			DataToSend[6].0 :=  iSSC2_Logic.0;
   			DataToSend[6].1 :=  iSSC2_Logic.1;
   			DataToSend[6].2 :=  iSSC2_Logic.2;
   			DataToSend[6].3 :=  iSSC2_Logic.3;
   			DataToSend[6].4 :=  iSSC2_Logic.4;
   			DataToSend[6].5 :=  iSSC2_Logic.5;
   			DataToSend[6].6 :=  iSSC2_Logic.6;
   			DataToSend[6].7 :=  iSSC2_Logic.7;
   
   			// Logic of the switch output 2, 0 = Deactivated, 1 = Single point, 2 = Window, 3 = Two point
   			DataToSend[6].8 :=  iSSC2_Mode.0;
   			DataToSend[6].9 :=  iSSC2_Mode.1;
   			DataToSend[6].10 := iSSC2_Mode.2;
   			DataToSend[6].11 := iSSC2_Mode.3;
   			DataToSend[6].12 := iSSC2_Mode.4;
   			DataToSend[6].13 := iSSC2_Mode.5;
   			DataToSend[6].14 := iSSC2_Mode.6;
   			DataToSend[6].15 := iSSC2_Mode.7;
   
   			// Hysteresis
   			COP(iSSC2_Hysteresis,SimulationDINT,1);		// Copy the Bits from the Real in a DINT
   
   			DataToSend[7].0 :=  SimulationDINT.24;
   			DataToSend[7].1 :=  SimulationDINT.25;
   			DataToSend[7].2 :=  SimulationDINT.26;
   			DataToSend[7].3 :=  SimulationDINT.27;
   			DataToSend[7].4 :=  SimulationDINT.28;
   			DataToSend[7].5 :=  SimulationDINT.29;
   			DataToSend[7].6 :=  SimulationDINT.30;
   			DataToSend[7].7 :=  SimulationDINT.31;
   			DataToSend[7].8 :=  SimulationDINT.16;
   			DataToSend[7].9 :=  SimulationDINT.17;
   			DataToSend[7].10 := SimulationDINT.18;
   			DataToSend[7].11 := SimulationDINT.19;
   			DataToSend[7].12 := SimulationDINT.20;
   			DataToSend[7].13 := SimulationDINT.21;
   			DataToSend[7].14 := SimulationDINT.22;
   			DataToSend[7].15 := SimulationDINT.23;
   			DataToSend[8].0  := SimulationDINT.8;
   			DataToSend[8].1  := SimulationDINT.9;
   			DataToSend[8].2  := SimulationDINT.10;
   			DataToSend[8].3  := SimulationDINT.11;
   			DataToSend[8].4  := SimulationDINT.12;
   			DataToSend[8].5  := SimulationDINT.13;
   			DataToSend[8].6  := SimulationDINT.14;
   			DataToSend[8].7  := SimulationDINT.15;
   			DataToSend[8].8  := SimulationDINT.0;
   			DataToSend[8].9  := SimulationDINT.1;
   			DataToSend[8].10 := SimulationDINT.2;
   			DataToSend[8].11 := SimulationDINT.3;
   			DataToSend[8].12 := SimulationDINT.4;
   			DataToSend[8].13 := SimulationDINT.5;
   			DataToSend[8].14 := SimulationDINT.6;
   			DataToSend[8].15 := SimulationDINT.7;
   
   			Trigger := TRUE;
   
   			if DeviceData.NewState then
   
   				DeviceData.StateDone := TRUE;
   
   			end_if;
   
   			if DeviceData.CommSuccess and DeviceData.ReplayIndex = CMD_Index then
   
   				Trigger := FALSE;
   				DeviceData.OldState := DeviceData.State;
   				DeviceData.State := DeviceData.State + 1;
   				DeviceData.CommSuccess := FALSE;
   				DeviceData.AcyclicData[0] := 0;
   				DeviceData.NewState := TRUE;
   
   			elsif DeviceData.CommTimeOut then
   
   				temp_string1 := 'Error in step ';
   				Temp_DINT := DeviceData.State;
   				DTOS(Temp_DINT, temp_string2);
   				CONCAT(temp_string1, temp_string2, qAOI_Diagnostic_String);
   
   				DeviceData.OldState := DeviceData.State;
   				DeviceData.State := DeviceData.MaxState;	//Check State
   				DeviceData.CommTimeOut := FALSE;
   				DeviceData.AcyclicData[0] := 0;
   				DeviceData.NewState := TRUE;
   
   			end_if;
   
   		//****************************************
   		47: // Read back set points SSC1 SetPoints
   		//****************************************
   			CMD_Index := 60;
   			CMD_Subindex := 0;
   			CMD_Wr := FALSE;
   			CMD_Rd := TRUE;
   			CMD_ByteLength := 8;
   
   			Trigger := TRUE;
   
   			if DeviceData.NewState then
   
   				DeviceData.StateDone := TRUE;
   
   			end_if;
   
   			if DeviceData.CommSuccess and DeviceData.ReplayIndex = CMD_Index then
   
   				// SetPoint1
   			 	COP(DeviceData.AcyclicData[0], qSSC1_SetPoint1,1);		// Copy the Bits from the Real in a DINT
   
   				// SetPoint2
   				COP(DeviceData.AcyclicData[1], qSSC1_SetPoint2,1);		// Copy the Bits from the Real in a DINT
   
   				Trigger := FALSE;
   				DeviceData.OldState := DeviceData.State;
   				DeviceData.State := DeviceData.State + 1;
   				DeviceData.CommSuccess := FALSE;
   				DeviceData.AcyclicData[0] := 0;
   				DeviceData.NewState := TRUE;
   
   			elsif DeviceData.CommTimeOut then
   
   				temp_string1 := 'Error in step ';
   				Temp_DINT := DeviceData.State;
   				DTOS(Temp_DINT, temp_string2);
   				CONCAT(temp_string1, temp_string2, qAOI_Diagnostic_String);
   
   				DeviceData.OldState := DeviceData.State;
   				DeviceData.State := DeviceData.MaxState;	//Check State
   				DeviceData.CommTimeOut := FALSE;
   				DeviceData.AcyclicData[0] := 0;
   				DeviceData.NewState := TRUE;
   
   			end_if;
   
   
   		//****************************************
   		48: // Read back set points SSC2 SetPoints
   		//****************************************
   			CMD_Index := 62;
   			CMD_Subindex := 0;
   			CMD_Wr := FALSE;
   			CMD_Rd := TRUE;
   			CMD_ByteLength := 8;
   
   			Trigger := TRUE;
   
   			if DeviceData.NewState then
   
   				DeviceData.StateDone := TRUE;
   
   			end_if;
   
   			if DeviceData.CommSuccess and DeviceData.ReplayIndex = CMD_Index then
   
   				// SetPoint1
   			 	COP(DeviceData.AcyclicData[0], qSSC2_SetPoint1,1);		// Copy the Bits from the Real in a DINT
   
   				// SetPoint2
   				COP(DeviceData.AcyclicData[1], qSSC2_SetPoint2,1);		// Copy the Bits from the Real in a DINT
   
   				Trigger := FALSE;
   				DeviceData.OldState := DeviceData.State;
   				DeviceData.State := DeviceData.MaxState;
   				DeviceData.CommSuccess := FALSE;
   				DeviceData.AcyclicData[0] := 0;
   				DeviceData.NewState := TRUE;
   
   			elsif DeviceData.CommTimeOut then
   
   				temp_string1 := 'Error in step ';
   				Temp_DINT := DeviceData.State;
   				DTOS(Temp_DINT, temp_string2);
   				CONCAT(temp_string1, temp_string2, qAOI_Diagnostic_String);
   
   				DeviceData.OldState := DeviceData.State;
   				DeviceData.State := DeviceData.MaxState;	//Check State
   				DeviceData.CommTimeOut := FALSE;
   				DeviceData.AcyclicData[0] := 0;
   				DeviceData.NewState := TRUE;
   
   			end_if;
   
   		//*********************************
   		50: // Teach SSC1
   		//*********************************
   
   			CMD_Index := 58;
   			CMD_Subindex := 0;
   			CMD_Wr := TRUE;
   			CMD_Rd := FALSE;
   			CMD_ByteLength := 1;
   
   			//Trigger to teach SSC1
   			DataToSend[6] :=  1;
   
   			Trigger := TRUE;
   
   			if DeviceData.NewState then
   
   				DeviceData.StateDone := TRUE;
   
   			end_if;
   
   			if DeviceData.CommSuccess and DeviceData.ReplayIndex = CMD_Index then
   
   				Trigger := FALSE;
   				DeviceData.OldState := DeviceData.State;
   				DeviceData.State := DeviceData.State + 1;
   				DeviceData.CommSuccess := FALSE;
   				DeviceData.AcyclicData[0] := 0;
   				DeviceData.NewState := TRUE;
   
   			elsif DeviceData.CommTimeOut then
   
   				temp_string1 := 'Error in step ';
   				Temp_DINT := DeviceData.State;
   				DTOS(Temp_DINT, temp_string2);
   				CONCAT(temp_string1, temp_string2, qAOI_Diagnostic_String);
   
   				DeviceData.OldState := DeviceData.State;
   				DeviceData.State := DeviceData.MaxState;	//Check State
   				DeviceData.CommTimeOut := FALSE;
   				DeviceData.AcyclicData[0] := 0;
   				DeviceData.NewState := TRUE;
   
   			end_if;
   
   		//*********************************
   		51: // Intermediate state
   		//*********************************
   
   			TONR (StandardTimer);
   			StandardTimer.PRE := 1000;
   			StandardTimer.TimerEnable := DeviceData.NewState;
   
   			if StandardTimer.DN then
   
   				DeviceData.OldState := DeviceData.State;
   				DeviceData.State := DeviceData.State + 1;
   
   			end_if;
   
   		//*********************************
   		52: // System command teach
   		//*********************************
   
   			CMD_Index := 2;
   			CMD_Subindex := 0;
   			CMD_Wr := TRUE;
   			CMD_Rd := FALSE;
   			CMD_ByteLength := 1;
   
   			// Selection of the setpoint of SSC1, 1 = Set point 1, 2 = Set point 2
   			if iSelectSP_SSC1 = 1 then
   
   				DataToSend[6] :=  65;
   
   			elsif iSelectSP_SSC1 = 2 then
   
   				DataToSend[6] :=  66;
   
   			end_if;
   
   			Trigger := TRUE;
   
   			if DeviceData.NewState then
   
   				DeviceData.StateDone := TRUE;
   
   			end_if;
   
   			if DeviceData.CommSuccess and DeviceData.ReplayIndex = CMD_Index then
   
   				Trigger := FALSE;
   				DeviceData.OldState := DeviceData.State;
   				DeviceData.State := DeviceData.State + 1;
   				DeviceData.CommSuccess := FALSE;
   				DeviceData.AcyclicData[0] := 0;
   				DeviceData.NewState := TRUE;
   
   			elsif DeviceData.CommTimeOut then
   
   				temp_string1 := 'Error in step ';
   				Temp_DINT := DeviceData.State;
   				DTOS(Temp_DINT, temp_string2);
   				CONCAT(temp_string1, temp_string2, qAOI_Diagnostic_String);
   
   				DeviceData.OldState := DeviceData.State;
   				DeviceData.State := DeviceData.MaxState;	//Check State
   				DeviceData.CommTimeOut := FALSE;
   				DeviceData.AcyclicData[0] := 0;
   				DeviceData.NewState := TRUE;
   
   			end_if;
   
   		//*********************************
   		53: // Intermediate state
   		//*********************************
   
   			StandardTimer.PRE := 1000;
   			StandardTimer.TimerEnable := DeviceData.NewState;
   
   			if StandardTimer.DN then
   
   				DeviceData.OldState := DeviceData.State;
   				DeviceData.State := DeviceData.State + 1;
   
   			end_if;
   
   		//****************************************
   		54: // Read back set points SSC1
   		//****************************************
   			CMD_Index := 60;
   			CMD_Subindex := 0;
   			CMD_Wr := FALSE;
   			CMD_Rd := TRUE;
   			CMD_ByteLength := 8;
   
   			Trigger := TRUE;
   
   			if DeviceData.NewState then
   
   				DeviceData.StateDone := TRUE;
   
   			end_if;
   
   			if DeviceData.CommSuccess and DeviceData.ReplayIndex = CMD_Index then
   
   				// SetPoint1
   			 	COP(DeviceData.AcyclicData[0], qSSC1_SetPoint1,1);		// Copy the Bits from the Real in a DINT
   
   				// SetPoint2
   				COP(DeviceData.AcyclicData[1], qSSC1_SetPoint2,1);		// Copy the Bits from the Real in a DINT
   
   				Trigger := FALSE;
   				DeviceData.OldState := DeviceData.State;
   				DeviceData.State := DeviceData.MaxState;
   				DeviceData.CommSuccess := FALSE;
   				DeviceData.AcyclicData[0] := 0;
   				DeviceData.NewState := TRUE;
   
   			elsif DeviceData.CommTimeOut then
   
   				temp_string1 := 'Error in step ';
   				Temp_DINT := DeviceData.State;
   				DTOS(Temp_DINT, temp_string2);
   				CONCAT(temp_string1, temp_string2, qAOI_Diagnostic_String);
   
   				DeviceData.OldState := DeviceData.State;
   				DeviceData.State := DeviceData.MaxState;	//Check State
   				DeviceData.CommTimeOut := FALSE;
   				DeviceData.AcyclicData[0] := 0;
   				DeviceData.NewState := TRUE;
   
   			end_if;
   
   		//*********************************
   		60: // Teach SSC2
   		//*********************************
   
   			CMD_Index := 58;
   			CMD_Subindex := 0;
   			CMD_Wr := TRUE;
   			CMD_Rd := FALSE;
   			CMD_ByteLength := 1;
   
   			//Trigger to teach SSC2
   			DataToSend[6] :=  2;
   
   			Trigger := TRUE;
   
   			if DeviceData.NewState then
   
   				DeviceData.StateDone := TRUE;
   
   			end_if;
   
   			if DeviceData.CommSuccess and DeviceData.ReplayIndex = CMD_Index then
   
   				Trigger := FALSE;
   				DeviceData.OldState := DeviceData.State;
   				DeviceData.State := DeviceData.State + 1;
   				DeviceData.CommSuccess := FALSE;
   				DeviceData.AcyclicData[0] := 0;
   				DeviceData.NewState := TRUE;
   
   			elsif DeviceData.CommTimeOut then
   
   				temp_string1 := 'Error in step ';
   				Temp_DINT := DeviceData.State;
   				DTOS(Temp_DINT, temp_string2);
   				CONCAT(temp_string1, temp_string2, qAOI_Diagnostic_String);
   
   				DeviceData.OldState := DeviceData.State;
   				DeviceData.State := DeviceData.MaxState;	//Check State
   				DeviceData.CommTimeOut := FALSE;
   				DeviceData.AcyclicData[0] := 0;
   				DeviceData.NewState := TRUE;
   
   			end_if;
   
   
   
   		//*********************************
   		61: // Intermediate state
   		//*********************************
   
   			StandardTimer.PRE := 1000;
   			StandardTimer.TimerEnable := DeviceData.NewState;
   
   			if StandardTimer.DN then
   
   				DeviceData.OldState := DeviceData.State;
   				DeviceData.State := DeviceData.State + 1;
   
   			end_if;
   
   		//*********************************
   		62: // System command teach
   		//*********************************
   
   			CMD_Index := 2;
   			CMD_Subindex := 0;
   			CMD_Wr := TRUE;
   			CMD_Rd := FALSE;
   			CMD_ByteLength := 1;
   
   			// Selection of the setpoint of SSC2, 1 = Set point 1, 2 = Set point 2
   			if iSelectSP_SSC2 = 1 then
   
   				DataToSend[6] :=  65;
   
   			elsif iSelectSP_SSC2 = 2 then
   
   				DataToSend[6] :=  66;
   
   			end_if;
   
   			Trigger := TRUE;
   
   			if DeviceData.NewState then
   
   				DeviceData.StateDone := TRUE;
   
   			end_if;
   
   			if DeviceData.CommSuccess and DeviceData.ReplayIndex = CMD_Index then
   
   				Trigger := FALSE;
   				DeviceData.OldState := DeviceData.State;
   				DeviceData.State := DeviceData.State + 1;
   				DeviceData.CommSuccess := FALSE;
   				DeviceData.AcyclicData[0] := 0;
   				DeviceData.NewState := TRUE;
   
   			elsif DeviceData.CommTimeOut then
   
   				temp_string1 := 'Error in step ';
   				Temp_DINT := DeviceData.State;
   				DTOS(Temp_DINT, temp_string2);
   				CONCAT(temp_string1, temp_string2, qAOI_Diagnostic_String);
   
   				DeviceData.OldState := DeviceData.State;
   				DeviceData.State := DeviceData.MaxState;	//Check State
   				DeviceData.CommTimeOut := FALSE;
   				DeviceData.AcyclicData[0] := 0;
   				DeviceData.NewState := TRUE;
   
   			end_if;
   		//*********************************
   		63: // Intermediate state
   		//*********************************
   
   			StandardTimer.PRE := 1000;
   			StandardTimer.TimerEnable := DeviceData.NewState;
   
   			if StandardTimer.DN then
   
   				DeviceData.OldState := DeviceData.State;
   				DeviceData.State := DeviceData.State + 1;
   
   			end_if;
   
   		//*****************************************
   		64: // Read back set points SSC2
   		//*****************************************
   			CMD_Index := 62;
   			CMD_Subindex := 0;
   			CMD_Wr := FALSE;
   			CMD_Rd := TRUE;
   			CMD_ByteLength := 8;
   
   			Trigger := TRUE;
   
   			if DeviceData.NewState then
   
   				DeviceData.StateDone := TRUE;
   
   			end_if;
   
   			if DeviceData.CommSuccess and DeviceData.ReplayIndex = CMD_Index then
   
   				// SetPoint1
   			 	COP(DeviceData.AcyclicData[0], qSSC2_SetPoint1,1);		// Copy the Bits from the Real in a DINT
   
   				// SetPoint2
   				COP(DeviceData.AcyclicData[1], qSSC2_SetPoint2,1);		// Copy the Bits from the Real in a DINT
   
   				Trigger := FALSE;
   
   				DeviceData.OldState := DeviceData.State;
   				DeviceData.State := DeviceData.MaxState;
   				DeviceData.CommSuccess := FALSE;
   				DeviceData.AcyclicData[0] := 0;
   				DeviceData.NewState := TRUE;
   
   			elsif DeviceData.CommTimeOut then
   
   				temp_string1 := 'Error in step ';
   				Temp_DINT := DeviceData.State;
   				DTOS(Temp_DINT, temp_string2);
   				CONCAT(temp_string1, temp_string2, qAOI_Diagnostic_String);
   
   				DeviceData.OldState := DeviceData.State;
   				DeviceData.State := DeviceData.MaxState;	//Check State
   				DeviceData.CommTimeOut := FALSE;
   				DeviceData.AcyclicData[0] := 0;
   				DeviceData.NewState := TRUE;
   
   			end_if;
   
   		//*********************************
   		90: // Actual Diagnostic
   		//*********************************
   
   			CMD_Index := 8284;
   			CMD_Subindex := 0;
   			CMD_Wr := FALSE;
   			CMD_Rd := TRUE;
   			CMD_ByteLength := 2;
   			Trigger := TRUE;
   
   			if DeviceData.NewState then
   
   				DeviceData.StateDone := TRUE;
   
   			end_if;
   
   			if  DeviceData.CommSuccess and DeviceData.ReplayIndex = CMD_Index then
   
   				qActual_Diagnostics_Code	:= DeviceData.AcyclicData[0];
   
   				case qActual_Diagnostics_Code of
   					0:
   			            qActual_Diagnostics_String := 'Device OK';
   			        4143:
   			            qActual_Diagnostics_String := 'S047 - Sensor limit reached';
   			        4897:
   			            qActual_Diagnostics_String := 'S801 - Supply voltage too low';
   			        4900:
   			            qActual_Diagnostics_String := 'S804 - Overload at switch output';
   			        4921:
   			            qActual_Diagnostics_String := 'S825 - Electronics temperature out of range';
   			        8593:
   			            qActual_Diagnostics_String := 'C401 - Factory reset active';
   			        8594:
   			            qActual_Diagnostics_String := 'C402 - Initialization active';
   			        8603:
   			            qActual_Diagnostics_String := 'C411 - Up-/download active';
   			        8677:
   			            qActual_Diagnostics_String := 'C485 - Process variable simulation active';
   			        8686:
   			            qActual_Diagnostics_String := 'C494 - Switch output simulation active';
   			        16425:
   			            qActual_Diagnostics_String := 'F041 - Sensor breakage detected';
   			        16427:
   			            qActual_Diagnostics_String := 'F043 - Sensor short circuit detected';
   			        16585:
   			            qActual_Diagnostics_String := 'F201 - Electronics faulty';
   			        16794:
   			            qActual_Diagnostics_String := 'F410 - Data transfer failed';
   			        16803:
   			            qActual_Diagnostics_String := 'F419 - Power cycle required';
   			        16921:
   			            qActual_Diagnostics_String := 'F537 - Configuration invalid';
   
   					else
   
   						qActual_Diagnostics_String := 'Error Code unknown';
   
   				end_case;
   
   			Trigger := FALSE;
   			DeviceData.OldState := DeviceData.State;
   			DeviceData.State := DeviceData.State + 1;
   			DeviceData.CommSuccess := FALSE;
   			DeviceData.AcyclicData[0] := 0;
   			DeviceData.NewState := TRUE;
   
   		elsif DeviceData.CommTimeOut then
   
   			temp_string1 := 'Error in step ';
   			Temp_DINT := DeviceData.State;
   			DTOS(Temp_DINT, temp_string2);
   			CONCAT(temp_string1, temp_string2, qAOI_Diagnostic_String);
   
   			DeviceData.OldState := DeviceData.State;
   			DeviceData.State := DeviceData.MaxState;
   			DeviceData.CommTimeOut := FALSE;
   			DeviceData.AcyclicData[0] := 0;
   			DeviceData.NewState := TRUE;
   
   		end_if;
   
   		//*********************************
   		91: // Last Diagnostic
   		//*********************************
   
   			CMD_Index := 8295;
   			CMD_Subindex := 0;
   			CMD_Wr := FALSE;
   			CMD_Rd := TRUE;
   			CMD_ByteLength := 2;
   			Trigger := TRUE;
   
   			if DeviceData.NewState then
   
   				DeviceData.StateDone := TRUE;
   
   			end_if;
   
   			if DeviceData.CommSuccess and DeviceData.ReplayIndex = CMD_Index then
   
   				qLast_Diagnostics_Code	:= DeviceData.AcyclicData[0];
   
   				case qLast_Diagnostics_Code of
   					0:
   			            qLast_Diagnostics_String := 'Device OK';
   			        4143:
   			            qLast_Diagnostics_String := 'S047 - Sensor limit reached';
   			        4897:
   			            qLast_Diagnostics_String := 'S801 - Supply voltage too low';
   			        4900:
   			            qLast_Diagnostics_String := 'S804 - Overload at switch output';
   			        4921:
   			            qLast_Diagnostics_String := 'S825 - Electronics temperature out of range';
   			        8593:
   			            qLast_Diagnostics_String := 'C401 - Factory reset active';
   			        8594:
   			            qLast_Diagnostics_String := 'C402 - Initialization active';
   			        8603:
   			            qLast_Diagnostics_String := 'C411 - Up-/download active';
   			        8677:
   			            qLast_Diagnostics_String := 'C485 - Process variable simulation active';
   			        8686:
   			            qLast_Diagnostics_String := 'C494 - Switch output simulation active';
   			        16425:
   			            qLast_Diagnostics_String := 'F041 - Sensor breakage detected';
   			        16427:
   			            qLast_Diagnostics_String := 'F043 - Sensor short circuit detected';
   			        16585:
   			            qLast_Diagnostics_String := 'F201 - Electronics faulty';
   			        16794:
   			            qLast_Diagnostics_String := 'F410 - Data transfer failed';
   			        16803:
   			            qLast_Diagnostics_String := 'F419 - Power cycle required';
   			        16921:
   			            qLast_Diagnostics_String := 'F537 - Configuration invalid';
   
   					else
   
   						qLast_Diagnostics_String := 'Error Code unknown';
   
   				end_case;
   
   				Trigger := FALSE;
   				DeviceData.OldState := DeviceData.State;
   				DeviceData.State := DeviceData.MaxState;
   				DeviceData.CommSuccess := FALSE;
   				DeviceData.AcyclicData[0] := 0;
   				DeviceData.NewState := TRUE;
   
   			elsif DeviceData.CommTimeOut then
   
   				temp_string1 := 'Error in step ';
   				Temp_DINT := DeviceData.State;
   				DTOS(Temp_DINT, temp_string2);
   				CONCAT(temp_string1, temp_string2, qAOI_Diagnostic_String);
   
   				DeviceData.OldState := DeviceData.State;
   				DeviceData.State := DeviceData.MaxState;    // Check State
   				DeviceData.CommTimeOut := FALSE;
   				DeviceData.AcyclicData[0] := 0;
   				DeviceData.NewState := TRUE;
   
   			end_if;
   
   		//*********************************
   		98: // End Step Trigger Guard
   		//*********************************
   
   			DeviceData.State := 0;
   			CommAOIBusy := 0;
   			DeviceAOISendRequest.[DeviceData.DevicePort] := 0;
   			ActiveComPort := 0;
   			ActiveAOI := 0;
   			DataToSend[0] := 0;
   			DataToSend[1] := 0;
   			DataToSend[2] := 0;
   			DataToSend[3] := 0;
   			DataToSend[4] := 0;
   			DataToSend[5] := 0;
    			DataToSend[6] := 0;
   			DataToSend[7] := 0;
   			DataToSend[8] := 0;
   			DataToSend[9] := 0;
   			DeviceData.StateDone := FALSE;
   			Skip := 0;
   			DeviceData.State := 0;
   			firstTimeDone := FALSE;
   			DeviceData.NewState := FALSE;
   			DeviceData.OldState := 0;
   			ActiveAOI := FALSE;
   
   			if SimActive then
   
   				SimActive := FALSE;
   				SimChanged := FALSE;
   
   			elsif UnitActive then
   
   				UnitActive := FALSE;
   				UnitChanged := FALSE;
   
   			elsif TeachSSC1TriggerActive then
   
   				TeachSSC1TriggerActive := FALSE;
   				TeachSSC1TriggerChanged := FALSE;
   
   			elsif TeachSSC2TriggerActive then
   
   				TeachSSC2TriggerActive := FALSE;
   				TeachSSC2TriggerChanged := FALSE;
   
   			elsif ParameterizeActive then
   
   				ParameterizeActive := FALSE;
   				ParameterizeChanged := FALSE;
   
   			elsif CondStatusActive then
   
   				CondStatusActive := FALSE;
   				CondStatusChanged := FALSE;
   
   			end_if;
   
   	end_case;
   
   	end_if;
   
   	//*************************
   	// Execution Area
   	//*************************
   
   	if DeviceData.State > StateMin and DeviceData.State < DeviceData.MaxState then
   
   		DataToSend[2] := DeviceData.DevicePort;
   		DataToSend[3] := CMD_Index;
   		DataToSend[4] := CMD_Subindex;
   		DataToSend[5].0 := CMD_Rd;
   		DataToSend[5].1 := CMD_Wr;
   		DataToSend[5].8 := CMD_ByteLength.0;  // Bits for the Length of the Data
   		DataToSend[5].9 := CMD_ByteLength.1;
   		DataToSend[5].10 := CMD_ByteLength.2;
   		DataToSend[5].11 := CMD_ByteLength.3;
   		DataToSend[5].12 := CMD_ByteLength.4;
   		DataToSend[5].13 := CMD_ByteLength.5;
   		DataToSend[5].14 := CMD_ByteLength.6;
   		DataToSend[5].15 := CMD_ByteLength.7;
   		DataToSend[5].7 := Trigger;
   
   		qCommError := CommError;
   
   	end_if;
   
   end_if;
END_ROUTINE
END_ADD_ON_INSTRUCTION
